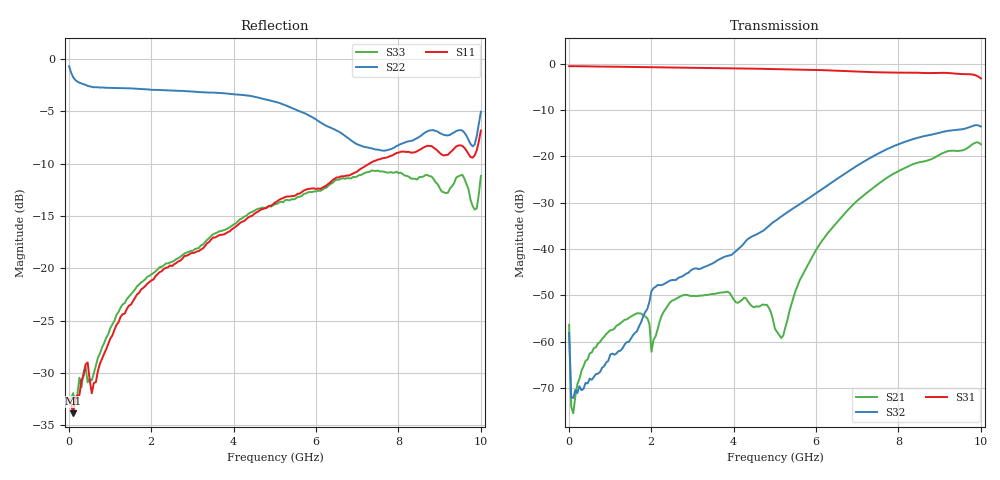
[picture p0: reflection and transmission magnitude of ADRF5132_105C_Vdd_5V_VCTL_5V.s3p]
! Device:  ADRF5132
! Description: Silicon SPDT Switch
! Frequency:  0.7 -  5 GHz
! Ports:
!	RFC	= Port 1
!	RF1	= Port 2
!  RF2  = Port 3
! Vdd:  5 Volt
! Control:  0/5 Volt
! Data:  Data was collected using a calibrated 4 port network analyzer and de-embedded using AtaiTec's In Situ De-Embedding.
! Note:  Analog Devices supplies this data as a sample of measured data
!  for this product.  Your particular data for this product may vary.
!  Data was taken at 105 degrees C.
!  Analog Devices reserves the right to change this data at anytime.
# GHZ S DB R 50.0
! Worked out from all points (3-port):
!   201 points, 10 MHz to 10 GHz, reference 50 ohm
!   strongest paths, dB at 10 MHz, 2.507 GHz, 5.005 GHz, 7.503 GHz, 10 GHz:
!     S31: -0.5, -0.8, -1.1, -1.8, -3.1
!     S32: -58.1, -46.7, -33.9, -19.4, -13.5
!     S21: -56.4, -51.2, -57.3, -26.0, -17.4
!   lowest |S11| = -33.9 dB at 109.9 MHz (marker M1), VSWR 1.04, Z = 52 - j0.492 ohm
!   |S11| at or under -10 dB: start of sweep to 7.301 GHz
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0.01  -32.53 -11.0  -56.89 -59.0  -0.49 -0.1
      -56.37 -58.0  -0.70 -8.1  -58.15 -58.3
      -0.48 -0.2  -58.11 -63.3  -32.75 19.1
0.05995  -33.01 -9.4  -74.73 -33.4  -0.50 -1.0
         -74.01 -23.7  -1.34 -42.5  -72.54 -38.3
         -0.49 -1.1  -72.01 -31.9  -32.41 -8.2
0.1099  -33.86 -13.5  -75.14 21.3  -0.50 -1.8
        -75.50 24.2  -1.76 -69.1  -72.14 -18.5
        -0.49 -1.9  -72.20 -17.5  -31.93 -13.6
0.35965  -30.29 -37.4  -65.87 66.5  -0.51 -5.8
         -65.33 60.9  -2.42 -135.5  -69.34 -35.7
         -0.51 -5.9  -70.23 -40.6  -29.96 -42.8
0.8092  -28.65 -70.7  -59.33 71.8  -0.57 -12.8
        -59.39 71.9  -2.73 -166.8  -65.98 -92.0
        -0.57 -12.8  -65.67 -91.2  -27.57 -61.9
3.85615  -16.56 -174.7  -49.23 71.8  -0.93 -59.1
         -49.20 72.3  -3.34 137.6  -41.48 177.4
         -0.93 -59.1  -41.48 177.5  -16.22 -123.2
5.005  -13.73 161.9  -57.09 93.2  -1.12 -76.7
       -57.25 95.6  -4.09 119.5  -33.92 173.1
       -1.12 -76.6  -33.94 173.3  -13.88 -137.9
7.003  -10.76 127.9  -29.53 158.7  -1.63 -108.2
       -29.53 158.6  -8.17 103.9  -21.94 132.3
       -1.63 -108.0  -21.95 132.6  -11.21 -162.9
9.6004  -8.50 69.3  -18.56 62.5  -2.20 -149.7
        -18.54 62.5  -7.05 95.2  -14.00 45.9
        -2.20 -149.5  -14.01 46.1  -11.44 161.7
10  -6.86 30.2  -17.38 22.5  -3.14 -170.2
    -17.36 22.4  -5.05 25.9  -13.52 21.4
    -3.13 -170.0  -13.53 21.7  -11.19 113.5
